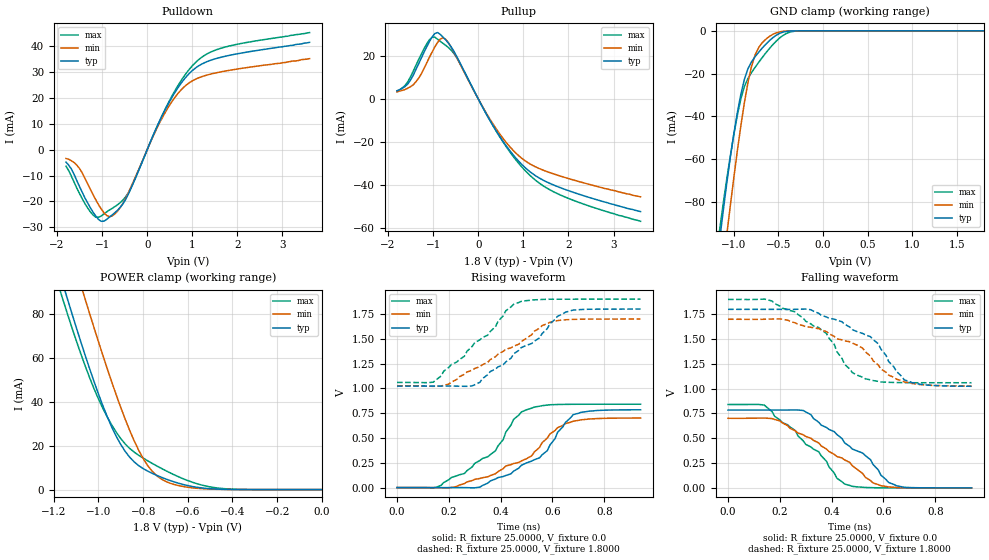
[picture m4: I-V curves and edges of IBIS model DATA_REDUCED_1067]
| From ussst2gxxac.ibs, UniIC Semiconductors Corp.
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|   Model DATA_REDUCED_1067
[Model]  DATA_REDUCED_1067
Model_type I/O
Polarity   Non-Inverting
Enable   Active-High
Vinl =   0.70000000V
Vinh =   1.10000000V
Vmeas =   0.90000000V
Rref =   25.00000000
Vref =   0.90000000V
C_comp   2.5240pF   2.5060pF   2.5510pF
[Temperature Range]   25.0000   95.0000   0.0
[Voltage Range]   1.8000V   1.7000V   1.9000V
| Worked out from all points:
|   slope of the pulldown table from 0 to 0.27 V, typ, clamps not added: 24.9 ohm
|   slope of the pullup table from 0 to 0.27 V, typ, clamps not added: 26.2 ohm
|   GND clamp passes 1 mA (typ) near -0.47 V on its own axis
|   POWER clamp passes 1 mA (typ) near -0.55 V on its own axis
|   rising waveform, R_fixture 25.0000, V_fixture 0.0: 20-80 % time 197ps typ, 222ps min, 178ps max; typ from 0 V to 0.784 V
|   rising waveform, R_fixture 25.0000, V_fixture 1.8000: 20-80 % time 221ps typ, 259ps min, 205ps max; typ from 1.02 V to 1.8 V
|   falling waveform, R_fixture 25.0000, V_fixture 0.0: 20-80 % time 221ps typ, 255ps min, 199ps max; typ from 0.784 V to 0 V
|   falling waveform, R_fixture 25.0000, V_fixture 1.8000: 20-80 % time 195ps typ, 227ps min, 178ps max; typ from 1.8 V to 1.02 V
[Pulldown]
|Voltage   I(typ)   I(min)   I(max)
-1.8V     -4.8mA     -3.4mA     -6.4mA
-1.5V     -14.3mA    -7.3mA     -17mA
-1.26V    -22.5mA    -15.4mA    -24.1mA
-1.14V    -25.73mA   -19.4mA    -26.15mA
-960mV    -27.7mA    -24.4mA    -24.93mA
-720mV    -24.45mA   -24.93mA   -22.1mA
-420mV    -17.33mA   -16.79mA   -16.77mA
420mV     16.17mA    15.06mA    16.48mA
720mV     24.99mA    22.57mA    25.9mA
1.02V     30.95mA    26.87mA    32.88mA
1.68V     36.02mA    30.33mA    39.55mA
3.6V      41.6mA     35.3mA     45.4mA
[Pullup]
|Voltage   I(typ)   I(min)   I(max)
-1.8V     3.7mA      3.2mA      3.6mA
-1.56V    6.9mA      4.9mA      7.9mA
-1.38V    13.6mA     7.9mA      15.5mA
-1.08V    26.53mA    19.24mA    27.32mA
-900mV    30.65mA    26.1mA     27.55mA
-780mV    28.58mA    28.2mA     25.65mA
-660mV    25.76mA    25.92mA    23.72mA
-420mV    17.3mA     16.82mA    17.01mA
360mV     -13.47mA   -12.68mA   -13.61mA
1.08V     -32.59mA   -29.26mA   -34.06mA
1.86V     -41.45mA   -36.02mA   -44.87mA
3.6V      -52.2mA    -45.4mA    -56.7mA
[GND_clamp]
|Voltage   I(typ)   I(min)   I(max)
-1.8V     -341.4mA   -368.9mA   -332.4mA
-1.16V    -98.84mA   -124.9mA   -94.02mA
-1.12V    -85.23mA   -110.5mA   -81.66mA
-1.08V    -72.2mA    -96.41mA   -70.06mA
-1.04V    -59.93mA   -82.62mA   -59.18mA
-920mV    -29.77mA   -44.48mA   -31.9mA
-880mV    -22.69mA   -33.57mA   -26.06mA
-800mV    -14.49mA   -16.62mA   -19.53mA
-720mV    -10.02mA   -7.817mA   -14.76mA
-560mV    -3.159mA   -1.628mA   -6.393mA
-280mV    -8.14uA    -3.578uA   -70uA
1.8V      7.234nA    32.16nA    61.22nA
[POWER_clamp]
|Voltage   I(typ)   I(min)   I(max)
-1.8V     325.1mA    352.4mA    316.2mA
-1.16V    94.14mA    121mA      86.98mA
-1.14V    87.41mA    114.1mA    80.57mA
-1.06V    61.46mA    87.09mA    56.62mA
-980mV    38.21mA    61.22mA    37.03mA
-900mV    20.56mA    37.47mA    23.27mA
-820mV    10.96mA    18mA       15.69mA
-780mV    8.467mA    11.05mA    13.18mA
-740mV    6.55mA     6.435mA    10.88mA
-640mV    2.87mA     1.791mA    5.795mA
-480mV    290.4uA    171.3uA    911.2uA
0V        7.234nA    10.13nA    70.66nA
[Ramp]
| variable   typ   min   max
dV/dt_r  0.4706/0.1900n  0.4209/0.2336n  0.5044/0.1772n
dV/dt_f  0.4656/0.1909n  0.4044/0.2349n  0.5040/0.1786n
R_load = 25.0000
[Rising Waveform]
R_fixture= 25.0000
V_fixture= 0.0
V_fixture_min= 0.0
V_fixture_max= 0.0
|time   V(typ)   V(min)   V(max)
0s        0V         0V         0V
150ps     -2.459uV   -597.8uV   2.441mV
260ps     -15.51uV   40.88mV    142.2mV
380ps     86.55mV    139.8mV    371.1mV
450ps     165.5mV    242.5mV    687.9mV
480ps     225.1mV    269.1mV    762.5mV
530ps     281.2mV    359.4mV    812.2mV
580ps     372.9mV    499.1mV    831.6mV
680ps     735.7mV    669.4mV    839.9mV
940ps     784.4mV    701.5mV    840.5mV
[Rising Waveform]
R_fixture= 25.0000
V_fixture= 1.8000
V_fixture_min= 1.7000
V_fixture_max= 1.9000
|time   V(typ)   V(min)   V(max)
0s        1.024V     1.026V     1.06V
140ps     1.024V     1.021V     1.063V
200ps     1.024V     1.044V     1.212V
290ps     1.025V     1.184V     1.423V
350ps     1.138V     1.263V     1.537V
420ps     1.267V     1.395V     1.783V
480ps     1.412V     1.473V     1.878V
560ps     1.553V     1.633V     1.897V
650ps     1.768V     1.692V     1.899V
940ps     1.8V       1.7V       1.9V
[Falling Waveform]
R_fixture= 25.0000
V_fixture= 0.0
V_fixture_min= 0.0
V_fixture_max= 0.0
|time   V(typ)   V(min)   V(max)
0s        784.4mV    701.5mV    840.6mV
140ps     784.4mV    703.8mV    834.9mV
200ps     784.4mV    675.6mV    685.2mV
290ps     780.2mV    535.4mV    475.2mV
350ps     662mV      453mV      363.8mV
450ps     453.6mV    281.7mV    38.55mV
560ps     235.1mV    49.36mV    1.549mV
620ps     53.83mV    9.269mV    158.9uV
650ps     21.65mV    4.043mV    64.38uV
940ps     2.342uV    1.515uV    0V
[Falling Waveform]
R_fixture= 25.0000
V_fixture= 1.8000
V_fixture_min= 1.7000
V_fixture_max= 1.9000
|time   V(typ)   V(min)   V(max)
0s        1.8V       1.7V       1.9V
150ps     1.8V       1.701V     1.899V
260ps     1.8V       1.663V     1.774V
320ps     1.796V     1.619V     1.653V
380ps     1.723V     1.575V     1.556V
450ps     1.65V      1.483V     1.245V
530ps     1.543V     1.372V     1.1V
580ps     1.453V     1.238V     1.073V
680ps     1.089V     1.069V     1.061V
940ps     1.024V     1.026V     1.06V
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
